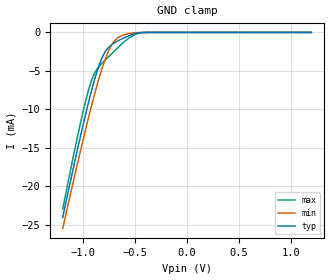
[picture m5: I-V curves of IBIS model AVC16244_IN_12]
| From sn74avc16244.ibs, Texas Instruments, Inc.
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[Model]   AVC16244_IN_12
Model_type  Input
Vinl=0
Vinh=1.2
| variable   typ   min   max
C_comp   3.88pF   3.07pF   4.71pF
[Temperature Range]   40   100   -40
| Ambient temperature   25   85   -40
[Voltage range]   1.2   1.2   1.2
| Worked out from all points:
|   GND clamp passes 1 mA (typ) near -0.65 V on its own axis
[GND Clamp]
| AVC16244_IN_12
|   Voltage   I(typ)   I(min)   I(max)
-1.2V     -24.05mA   -25.5mA    -22.96mA
-1.03V    -13.59mA   -15.46mA   -11.88mA
-970mV    -10.15mA   -12.11mA   -8.465mA
-925mV    -7.748mA   -9.701mA   -6.384mA
-875mV    -5.357mA   -7.175mA   -4.895mA
-840mV    -3.958mA   -5.541mA   -4.278mA
-805mV    -2.881mA   -4.063mA   -3.785mA
-740mV    -1.741mA   -1.926mA   -2.942mA
-675mV    -1.16mA    -781.6uA   -2.096mA
-545mV    -361.4uA   -112.5uA   -609.2uA
-430mV    -20.24uA   -13.73uA   -29.52uA
1.2V      195.2pA    673.5pA    10.43pA
